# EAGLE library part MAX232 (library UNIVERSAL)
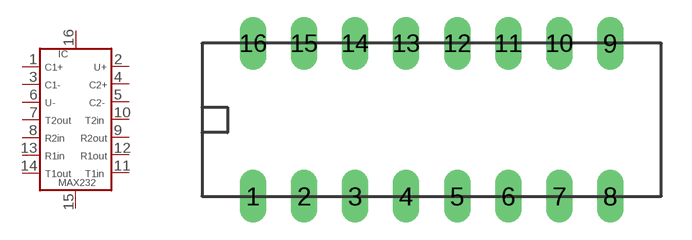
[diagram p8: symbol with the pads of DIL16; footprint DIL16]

Designator prefix IC

## MAX232  [DIL16]
1  1
2  2
3  3
4  4
5  5
6  6
7  7
8  8
9  9
10  10
11  11
12  12
13  13
14  14
15  15
16  16

## Footprint DIL16 (pad centres in mm)
drill 0.813 pad 1.27 long: 1 0,1.27; 2 2.54,1.27; 3 5.08,1.27; 4 7.62,1.27; 5 10.16,1.27; 6 12.7,1.27; 7 15.24,1.27; 8 17.78,1.27; 9 17.78,8.89; 10 15.24,8.89; 11 12.7,8.89; 12 10.16,8.89; 13 7.62,8.89; 14 5.08,8.89; 15 2.54,8.89; 16 0,8.89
